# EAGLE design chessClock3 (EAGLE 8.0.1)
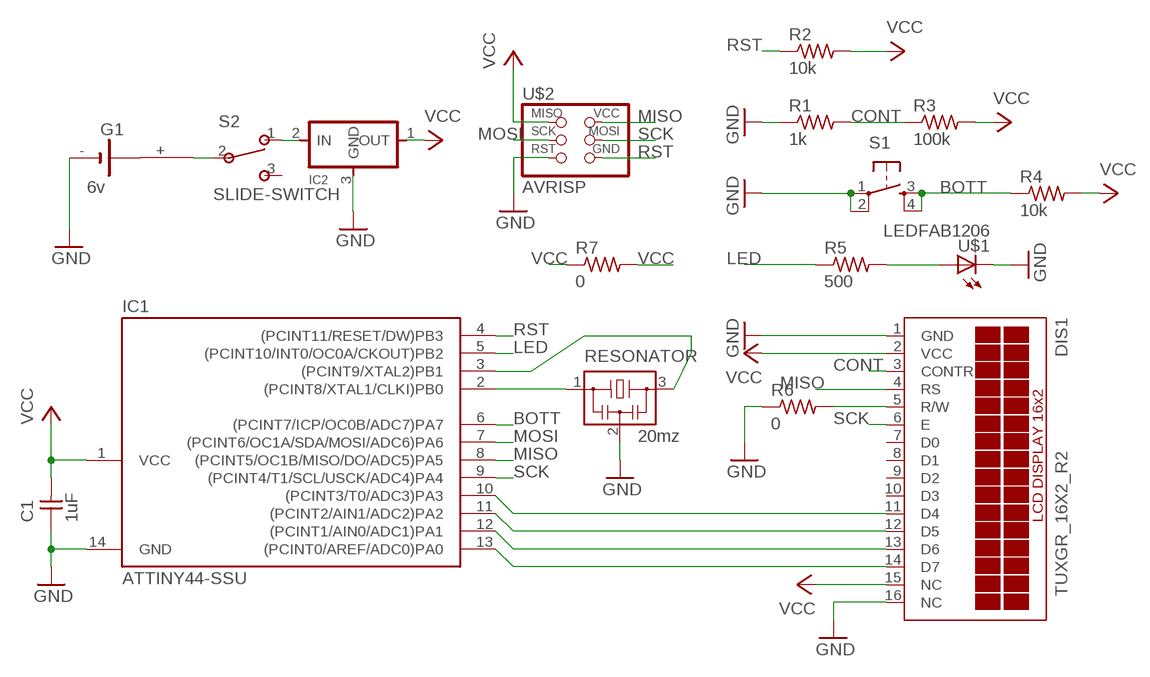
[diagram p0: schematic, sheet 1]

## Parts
C1  1uF  CAP-UNPOLARIZEDFAB  [C1206FAB]
DIS1  TUXGR_16X2_R2  [TUXGR_16X2_R2]
G1  6v  B2430UNI  [B2430UNI]
IC1  ATTINY44-SSU  [SOIC14]
IC2  REGULATORSOT23  [SOT23]
R1  1k  RES-US1206FAB  [R1206FAB]
R2  10k  RES-US1206FAB  [R1206FAB]
R3  100k  RES-US1206FAB  [R1206FAB]
R4  10k  RES-US1206FAB  [R1206FAB]
R5  500  RES-US1206FAB  [R1206FAB]
R6  0  RES-US1206FAB  [R1206FAB]
R7  0  RES-US1206FAB  [R1206FAB]
RESONATOR  20mz  RESONATOR  [EFOBM]
S1  6MM_SWITCH6MM_SWITCH  [6MM_SWITCH]
S2  SLIDE-SWITCH  [AYZ0102AGRLC]
U$1  LEDFAB1206  [LED1206FAB]
U$2  AVRISP  [2X03]

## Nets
BOTT: IC1.6((PCINT7/ICP/OC0B/ADC7)PA7) R4.1 S1.3(S) S1.4(S1)
CONT: DIS1.3(CONTR) R1.2 R3.1
GND: C1.1 DIS1.1(GND) DIS1.16(NC) G1.- IC1.14(GND) IC2.3(GND) R1.1 R6.1 RESONATOR.2 S1.1(P) S1.2(P1) U$1.2(C) U$2.5(RST)
LED: IC1.5((PCINT10/INT0/OC0A/CKOUT)PB2) R5.1
MISO: DIS1.4(RS) IC1.8((PCINT5/OC1B/MISO/DO/ADC5)PA5) U$2.2(VCC)
MOSI: IC1.7((PCINT6/OC1A/SDA/MOSI/ADC6)PA6) U$2.3(SCK)
N$1: IC1.3((PCINT9/XTAL2)PB1) RESONATOR.3
N$2: IC1.2((PCINT8/XTAL1/CLKI)PB0) RESONATOR.1
N$3: DIS1.14(D7) IC1.13((PCINT0/AREF/ADC0)PA0)
N$4: DIS1.13(D6) IC1.12((PCINT1/AIN0/ADC1)PA1)
N$5: DIS1.12(D5) IC1.11((PCINT2/AIN1/ADC2)PA2)
N$6: DIS1.11(D4) IC1.10((PCINT3/T0/ADC3)PA3)
N$7: G1.+ S2.2
N$10: R5.2 U$1.1(A)
N$11: DIS1.5(R/W) R6.2
N$12: IC2.2(IN) S2.1
RST: IC1.4((PCINT11/RESET/DW)PB3) R2.1 U$2.6(GND)
SCK: DIS1.6(E) IC1.9((PCINT4/T1/SCL/USCK/ADC4)PA4) U$2.4(MOSI)
VCC: C1.2 DIS1.2(VCC) DIS1.15(NC) IC1.1(VCC) IC2.1(OUT) R2.2 R3.2 R4.2 R7.1 R7.2 U$2.1(MISO)
Unconnected: DIS1.7(D0) DIS1.8(D1) DIS1.9(D2) DIS1.10(D3) G1.+@1(+) G1.+@2(+) G1.+@3(+) G1.+@4(+) G1.-@1(-) S2.3

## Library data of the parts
C1 = fab:CAP-UNPOLARIZED
DIS1 = display-lcd:TUXGR_16X2_R2: Tuxgraphics LCD display 16x2 characters reflective, without background light Source: tuxgr_12x2_r2.pdf; OC_FARNELL: unknown; OC_NEWARK: unknown
G1 = battery:B2430UNI: LI BATTERY
IC1 = fab:ATTINY44
IC2 = fab:REGULATOR
R1-R7 = fab:RES-US: Resistor (US Symbol)
RESONATOR = fab:RESONATOR
S1 = fab:6MM_SWITCH: OMRON SWITCH
S2 = fab:SLIDE-SWITCH: SMD slide-switch AYZ0102AGRLC as found in the fablab inventory. Includes the mounting holes. Made by Zaerc.
U$1 = fab:LED: LED
U$2 = fab:AVRISP

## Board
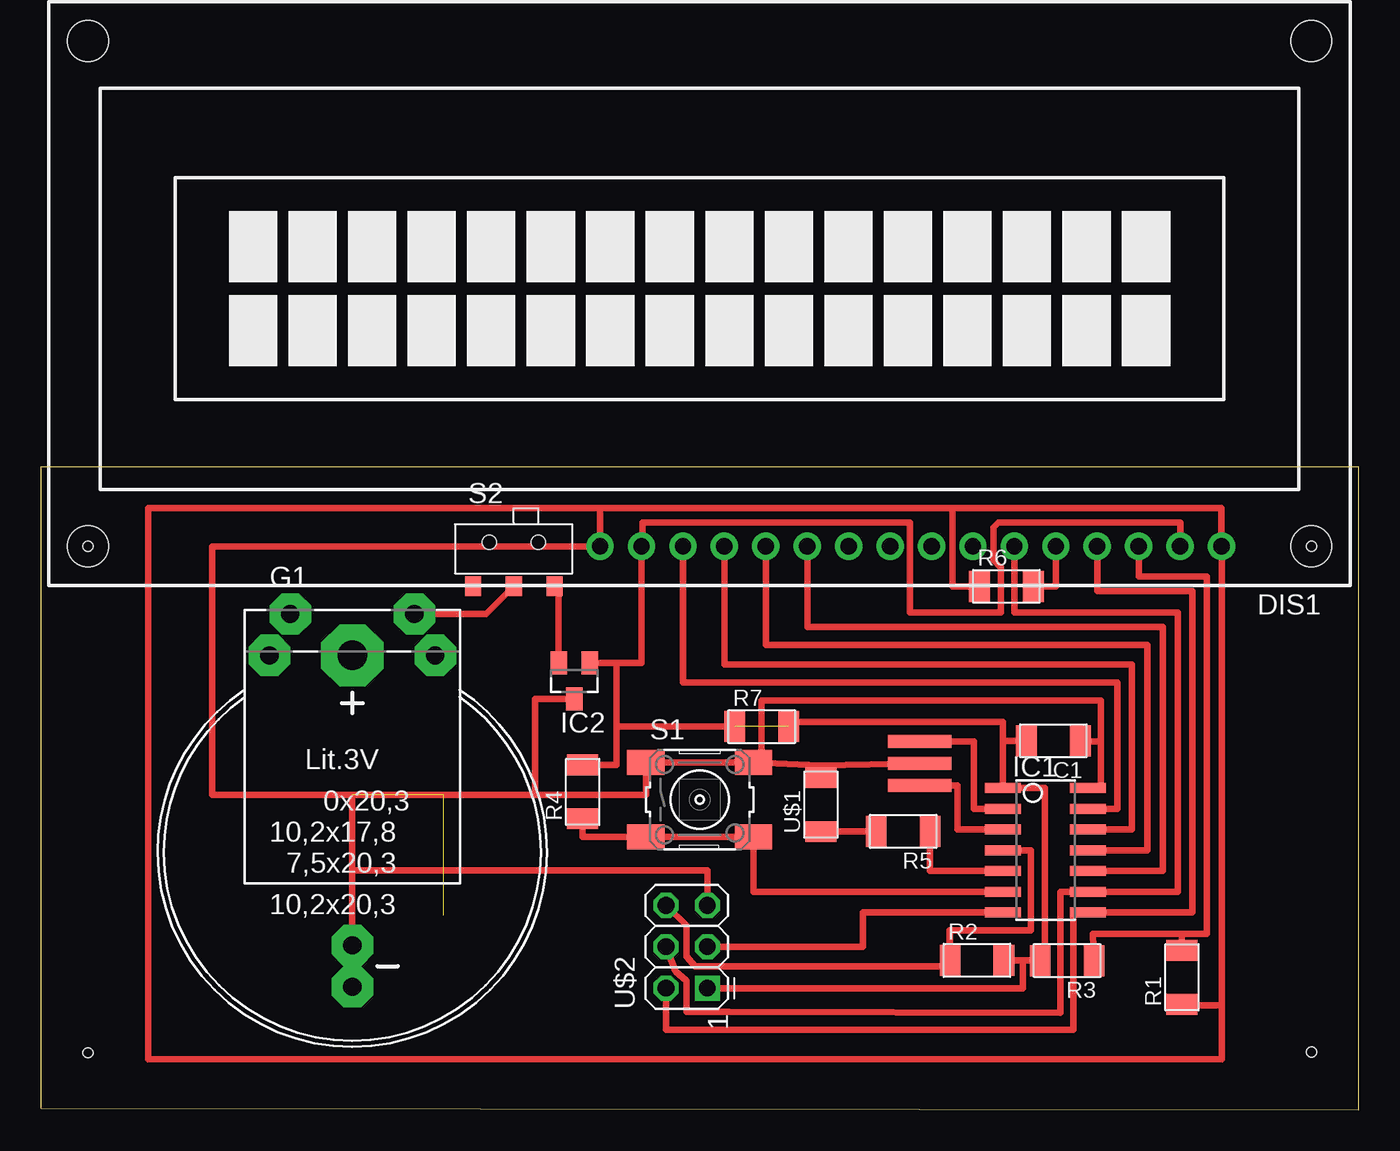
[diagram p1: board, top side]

Size 80.8 x 39.4 mm. Coordinates in mm from the lower left corner, seen from the top.
Outline: 0,0.1 0,39.4 80.8,39.4 80.8,0 0.03,0.1
Copper layers (1*16): Top 0.035mm / dielectric 1.5mm / Bottom 0.035mm
Design rules "default *": minimum track width 10mil, minimum drill 24mil, track to track 16mil, track to pad 8mil, pad to pad 8mil, via to via 8mil, smd to smd 1mil, copper to edge 24mil, drill to drill 8mil, minimum pad ring 10mil, minimum via ring 8mil, stop-mask expansion 0mil, vias tented up to drill 0mil, thermal gap 10mil
Holes 0.6 mm at 2.9,3.5 77.9,3.55 77.9,34.55 2.9,34.55

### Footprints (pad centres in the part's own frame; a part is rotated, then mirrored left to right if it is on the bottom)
C1206FAB = smd 1.27 x 1.905: 1 -1.651,0; 2 1.651,0
TUXGR_16X2_R2 = drill 1 pad 1.676: 1 -32,15.5; 2 -29.46,15.5; 3 -26.92,15.5; 4 -24.38,15.5; 5 -21.84,15.5; 6 -19.3,15.5; 7 -16.76,15.5; 8 -14.22,15.5; 9 -11.68,15.5; 10 -9.14,15.5; 11 -6.6,15.5; 12 -4.06,15.5; 13 -1.52,15.5; 14 1.02,15.5; 15 3.56,15.5; 16 6.1,15.5 | hole 2.5: -37.5,-15.5; 37.5,-15.5; -37.5,15.5; 37.5,15.5
B2430UNI = drill 1.118 pad 2.54 octagon: + 3.81,14.605; +@1 -3.81,14.605; +@2 -5.08,12.065; +@3 5.08,12.065; - 0,-5.715; -@1 0,-8.255 | drill 1.803 pad 3.81 octagon: +@4 0,12.065
SOIC14 = smd 0.61 x 2.21: 1 -3.81,-2.603; 2 -2.54,-2.603; 3 -1.27,-2.603; 4 0,-2.603; 5 1.27,-2.603; 6 2.54,-2.603; 7 3.81,-2.603; 8 3.81,2.603; 9 2.54,2.603; 10 1.27,2.603; 11 0,2.603; 12 -1.27,2.603; 13 -2.54,2.603; 14 -3.81,2.603
SOT23 = smd 1 x 1.4: 1 -0.95,-1.1; 2 0.95,-1.1; 3 0,1.1
R1206FAB = smd 1.27 x 1.905: 1 -1.651,0; 2 1.651,0
EFOBM = smd 0.8 x 3.9: 1 -1.35,0; 2 0,0; 3 1.35,0
6MM_SWITCH = smd 2.286 x 1.524: 1 -3.302,2.286; 2 3.302,2.286; 3 -3.302,-2.286; 4 3.302,-2.286
AYZ0102AGRLC = smd 1 x 1.2: 1 2.5,-2.3; 2 0,-2.3; 3 -2.5,-2.3 | hole 0.85: -1.5,0.4; 1.5,0.4
LED1206FAB = smd 1.27 x 1.905: 1 -1.651,0; 2 1.651,0
2X03 = drill 1.016 square: 1 -2.54,-1.27 | drill 1.016 octagon: 2 -2.54,1.27; 3 0,-1.27; 4 0,1.27; 5 2.54,-1.27; 6 2.54,1.27

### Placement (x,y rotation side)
C1  62.08,22.63 180 top
DIS1  40.39,50.05 180 top
G1  19.1,15.8 0 top
IC1  61.6,15.92 270 top
IC2  32.7,26.3 180 top
R1  69.96,8.13 90 top
R2  57.4,9.17 0 top
R3  62.92,9.15 180 top
R4  33.22,19.5 90 top
R5  52.88,17.08 180 top
R6  59.2,32.1 0 top
R7  44.2,23.5 0 top
RESONATOR  53.89,21.25 270 top
S1  40.4,19.03 0 top
S2  29,34.4 0 top
U$1  47.83,18.71 90 top
U$2  39.6,10 90 top

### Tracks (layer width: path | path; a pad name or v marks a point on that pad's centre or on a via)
BOTT
  Top 0.406: R4.1 33.22,16.74 S1.3 S1.4 43.7,13.38 IC1.6
CONT
  Top 0.406: DIS1.3 67.31,32.7 71.5,32.7 71.5,10.8 69.96,10.8 | 69.96,10.8 64.5,10.8 R3.1 | R1.2 69.96,10.8
GND  (2 unrouted)
  Top 0.406: S1.2 S1.1 37.09,19.3 30.3,19.3 | S1.2 44.19,21.07 44.18,25.1 63.2,25.1 | 34.29,36.9 DIS1.16 10.5,34.55 10.5,19.3 19.1,19.3 | 55.9,36.9 34.29,36.9 | 55.9,36.9 72.39,36.9 DIS1.1 72.4,34.65 72.4,6.4 | 63.2,25.1 63.5,25.1 | 47.8,21.12 RESONATOR.2 | 72.4,6.4 69.96,6.4 R1.1 | U$1.2 47.8,21.12 | IC2.3 30.3,25.2 30.3,19.3 | 19.1,14.7 19.1,19.3 | 19.1,14.7 G1.- | 19.1,19.3 30.3,19.3 | R6.1 55.9,32.1 55.9,36.9 | S1.2 47.8,21.12 | 63.2,25.1 65,25.1 65,22.6 | IC1.14 65,19.73 65,22.6 | C1.1 63.73,22.6 65,22.6 | 72.4,6.4 72.4,3.1 6.6,3.1 6.6,36.9 34.29,36.9 | U$2.5 40.87,14.7 19.1,14.7
LED
  Top 0.406: IC1.5 54.53,14.65 R5.1
MISO
  Top 0.406: DIS1.4 64.77,31.8 70.6,31.8 70.6,12.11 IC1.8 63.3,12.11 63.3,4.9 38.33,4.9 U$2.2
MOSI
  Top 0.406: IC1.7 50.4,12.11 50.4,10 U$2.3
N$1
  Top 0.406: IC1.3 56.2,17.2 56.2,19.9 RESONATOR.3
N$2
  Top 0.406: IC1.2 57.2,18.46 57.2,22.6 RESONATOR.1
N$3
  Top 0.406: DIS1.14 39.37,26.2 66,26.2 66,18.46 IC1.13
N$4
  Top 0.406: DIS1.13 41.91,27.3 66.9,27.3 66.9,17.19 IC1.12
N$5
  Top 0.406: DIS1.12 44.45,28.5 67.85,28.5 67.85,15.92 IC1.11
N$6
  Top 0.406: DIS1.11 46.99,29.6 68.8,29.6 68.8,14.65 IC1.10
N$7
  Top 0.406: S2.2 27.3,30.41 G1.+
N$10
  Top 0.406: R5.2 U$1.1
N$11
  Top 0.406: R6.2 62.23,32.1 DIS1.5
N$12
  Top 0.406: IC2.2 31.75,31.85 S2.1
RST
  Top 0.406: IC1.4 60.7,15.92 60.7,11 55.74,11 | 55.74,11 R2.1 | 55.74,11 55.7,11 55.7,8.8 40.1,8.8 39.6,9.4 39.6,11.3 U$2.6
SCK
  Top 0.406: DIS1.6 59.69,30.5 69.7,30.5 69.7,13.38 IC1.9 62.5,13.38 62.5,5.95 42.2,6 39.6,6 39.6,7.9 38.9,8.5 U$2.4
VCC  (1 unrouted)
  Top 0.406: DIS1.2 69.85,36 58.7,36 58.4,35.7 58.4,33.7 58.8,33.3 58.85,33.3 58.85,30.5 53.3,30.5 53.3,36 36.9,36 36.9,34.55 DIS1.15 36.83,27.4 35.3,27.4 | 59.33,19.73 IC1.1 | 59,22.63 C1.2 | 59,22.63 IC1.1 | IC1.1 61.55,19.73 61.55,9.43 arc-90 R3.2 arc90 61.25,9.17 60.2,9.17 | 35.3,27.4 IC2.1 | R4.2 35.3,21.15 35.3,23.5 | 35.3,23.5 35.3,27.4 | R7.1 35.3,23.5 | 59,22.63 59,23.8 45.85,23.8 R7.2 | 60.2,9.17 R2.2 | U$2.1 60.2,7.46 60.2,9.17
